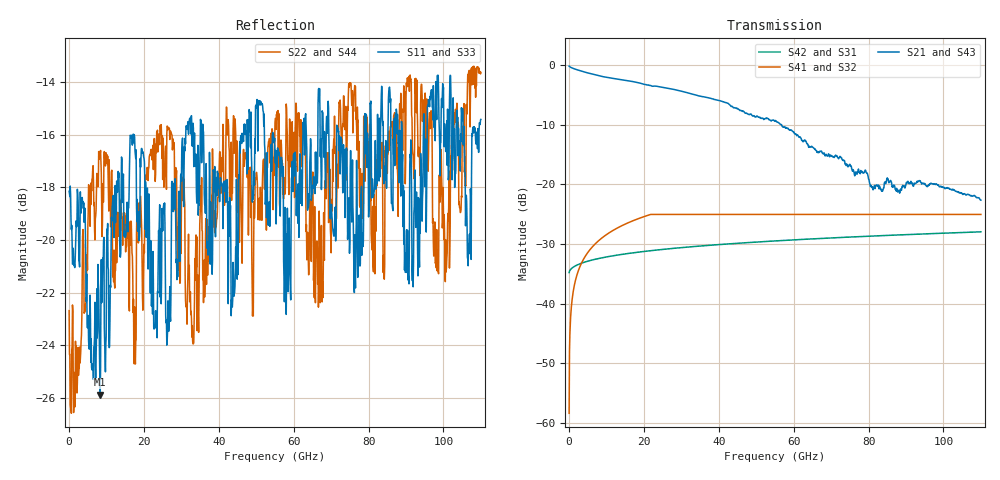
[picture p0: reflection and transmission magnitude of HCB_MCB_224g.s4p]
! Created with skrf 1.10.0 (http://scikit-rf.org).
# GHz S RI R 50.0
!freq ReS11 ImS11 ReS12 ImS12 ReS13 ImS13
! ReS14 ImS14
! ReS21 ImS21 ReS22 ImS22 ReS23 ImS23
! ReS24 ImS24
! ReS31 ImS31 ReS32 ImS32 ReS33 ImS33
! ReS34 ImS34
! ReS41 ImS41 ReS42 ImS42 ReS43 ImS43
! ReS44 ImS44
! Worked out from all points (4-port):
!   1101 points, 10 MHz to 110 GHz, reference 50 ohm
!   strongest paths, dB at 10 MHz, 27.51 GHz, 55.01 GHz, 82.5 GHz, 110 GHz:
!     S21: -0.2, -4.0, -9.4, -20.3, -22.6
!     S43: -0.2, -4.1, -9.4, -20.2, -22.6
!     S41: -58.4, -25.0, -25.0, -25.0, -25.0
!     S32: -58.4, -25.0, -25.0, -25.0, -25.0
!     S42: -34.8, -30.8, -29.5, -28.6, -28.0
!     S31: -34.8, -30.8, -29.5, -28.6, -28.0
!   lowest |S11| = -25.9 dB at 8.309 GHz (marker M1), VSWR 1.11, Z = 54.5 + j2.83 ohm
!   |S11| at or under -10 dB: start of sweep to end of sweep
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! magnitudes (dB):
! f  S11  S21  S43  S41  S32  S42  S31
! 10 MHz  -18.1  -0.2  -0.2  -58.4  -58.4  -34.8  -34.8
! 1.61 GHz  -20.8  -0.6  -0.7  -36.3  -36.3  -33.7  -33.7
! 8.309 GHz  -25.9  -1.8  -1.7  -29.2  -29.2  -32.4  -32.4
! 33.01 GHz  -15.8  -4.9  -4.8  -25.0  -25.0  -30.4  -30.4
! 42.31 GHz  -18.0  -6.4  -6.4  -25.0  -25.0  -30.0  -30.0
! 98.2 GHz  -15.4  -20.0  -19.9  -25.0  -25.0  -28.2  -28.2
! 110 GHz  -15.4  -22.6  -22.6  -25.0  -25.0  -28.0  -28.0
